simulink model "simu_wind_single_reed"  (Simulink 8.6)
settings: Solver=ode4  StartTime=0.0  StopTime=runtime  FixedStep=1/fs  RelTol=1e-3
PostLoadFcn:
  | , if any(exist('dsrtsu_mdlpostloadfcn', 'file') == [2, 3, 6]), try dsrtsu_mdlpostloadfcn('Execute', bdroot); catch fprintf('Error in PostLoadFcn (dsrtsu_mdlpostloadfcn) for model "%s":
  |  %s
  | ', bdroot, lasterr); end, end,
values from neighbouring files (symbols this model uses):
  an = modal_coeff(:,1)    [hybrid_wind.m]
  gamma_cte = 0.7    [single_reed.m]
  PM = 50    [bowed_string_hyperbolic.m]    (also in lip_reed.m = 20; single_reed.m = 100)
  Qn = modal_coeff(:,3)    [hybrid_wind.m]
  Ts = 25e-6    (= 2.5e-05)    [hybrid_wind.m]    (also in measurements.m)
  wn = modal_coeff(:,2)    [hybrid_wind.m]
  Zc = rho*c/St    (= 2615281.00417)    [hybrid_wind.m]
  zeta = 0.35    [single_reed.m]
undefined symbols (not defined in the file or in its folder): HRreed_G, HRreed_G_zm1, modal_coeff
libraries: simulink x1

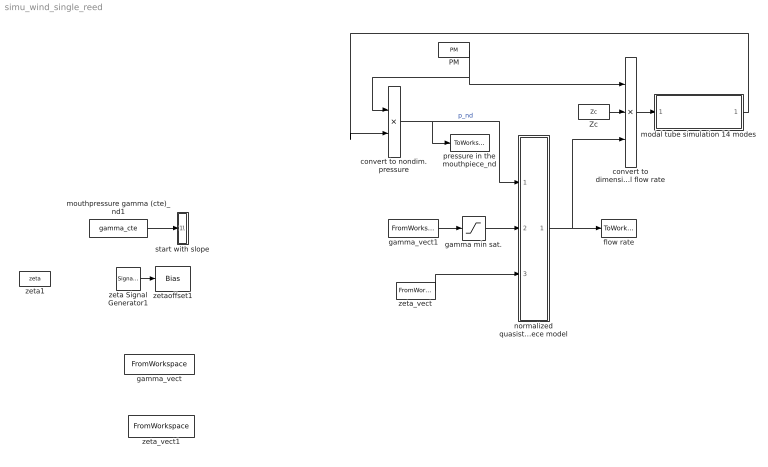
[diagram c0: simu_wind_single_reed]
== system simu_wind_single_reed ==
  PM : Constant  Value=PM
  Zc : Constant  Value=Zc
  convert to dimensional flow rate : Product  Inputs=*/*
  convert to nondim. pressure : Product  Inputs=/*
  flow rate : ToWorkspace  VariableName=q_dl  SaveFormat=Structure  SampleTime=-1
  gamma min sat. : Saturate  UpperLimit=100  LowerLimit=0.3
  gamma_vect : FromWorkspace  VariableName=gamma_envs_all  SampleTime=0
  gamma_vect1 : FromWorkspace  VariableName=gamma_vect  SampleTime=Ts  OutputAfterFinalValue=Setting to zero
  modal tube simulation 14 modes : Subsystem
  mouthpressure gamma (cte)_nd1 : Constant  Value=gamma_cte
  normalized quasistatic mouthpiece model : Subsystem
  pressure in the mouthpiece_nd : ToWorkspace  VariableName=p_dl  SaveFormat=Structure  SampleTime=-1
  start with slope : Subsystem
  zeta Signal Generator1 : SignalGenerator  WaveForm=sawtooth  Amplitude=(0.6-0.1)/2  Frequency=0.2
  zeta1 : Constant  Value=zeta
  zeta_vect : FromWorkspace  VariableName=zeta_vect  SampleTime=Ts  OutputAfterFinalValue=Setting to zero
  zeta_vect1 : FromWorkspace  VariableName=zeta_envs_all_a  SampleTime=0  OutputAfterFinalValue=Setting to zero
  zetaoffset1 : Bias  Bias=0.1+(0.6-0.1)/2
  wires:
  zeta Signal Generator1/1 -> zetaoffset1/1
  Zc/1 -> convert to dimensional flow rate/2
  PM/1 -> convert to nondim. pressure/1, convert to dimensional flow rate/1
  mouthpressure gamma (cte)_nd1/1 -> start with slope/1(gamma_in)
  convert to dimensional flow rate/1 -> modal tube simulation 14 modes/1(flowrate_in)
  modal tube simulation 14 modes/1(p_sim_out) -> convert to nondim. pressure/2
  gamma_vect1/1 -> gamma min sat./1
  gamma min sat./1 -> normalized quasistatic mouthpiece model/2(gamma)
  convert to nondim. pressure/1 -> pressure in the mouthpiece_nd/1, normalized quasistatic mouthpiece model/1(p)  "p_nd"
  normalized quasistatic mouthpiece model/1(q_nd) -> flow rate/1, convert to dimensional flow rate/3
  zeta_vect/1 -> normalized quasistatic mouthpiece model/3(zeta)

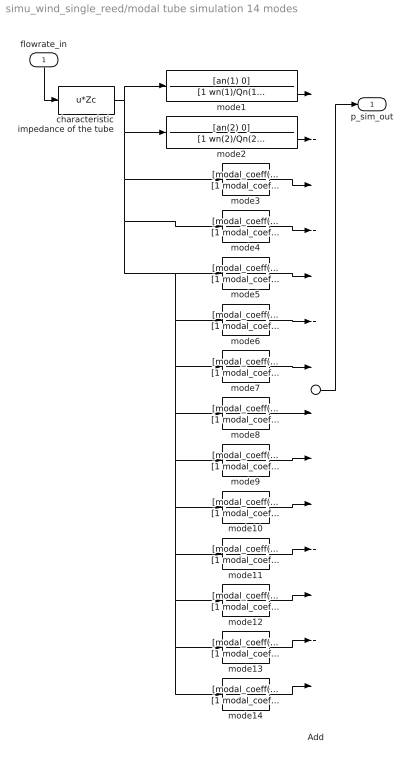
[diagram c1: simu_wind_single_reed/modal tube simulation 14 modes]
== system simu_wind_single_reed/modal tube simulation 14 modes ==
  flowrate_in : Inport
  Add : Sum  Inputs=++++++++++++++
  characteristic impedance of the tube : Fcn  Expr=u*Zc
  mode1 : TransferFcn  Numerator=[an(1) 0]  Denominator=[1 wn(1)/Qn(1) wn(1)^2]
  mode10 : TransferFcn  Numerator=[modal_coeff(10, 1) 0]  Denominator=[1 modal_coeff(10,2)/modal_coeff(10,3) modal_coeff(10,2)^2]
  mode11 : TransferFcn  Numerator=[modal_coeff(11, 1) 0]  Denominator=[1 modal_coeff(11,2)/modal_coeff(11,3) modal_coeff(11,2)^2]
  mode12 : TransferFcn  Numerator=[modal_coeff(12, 1) 0]  Denominator=[1 modal_coeff(12,2)/modal_coeff(12,3) modal_coeff(12,2)^2]
  mode13 : TransferFcn  Numerator=[modal_coeff(13, 1) 0]  Denominator=[1 modal_coeff(13,2)/modal_coeff(13,3) modal_coeff(13,2)^2]
  mode14 : TransferFcn  Numerator=[modal_coeff(14, 1) 0]  Denominator=[1 modal_coeff(14,2)/modal_coeff(14,3) modal_coeff(14,2)^2]
  mode2 : TransferFcn  Numerator=[an(2) 0]  Denominator=[1 wn(2)/Qn(2) wn(2)^2]
  mode3 : TransferFcn  Numerator=[modal_coeff(3, 1) 0]  Denominator=[1 modal_coeff(3,2)/modal_coeff(3,3) modal_coeff(3,2)^2]
  mode4 : TransferFcn  Numerator=[modal_coeff(4, 1) 0]  Denominator=[1 modal_coeff(4,2)/modal_coeff(4,3) modal_coeff(4,2)^2]
  mode5 : TransferFcn  Numerator=[modal_coeff(5, 1) 0]  Denominator=[1 modal_coeff(5,2)/modal_coeff(5,3) modal_coeff(5,2)^2]
  mode6 : TransferFcn  Numerator=[modal_coeff(6, 1) 0]  Denominator=[1 modal_coeff(6,2)/modal_coeff(6,3) modal_coeff(6,2)^2]
  mode7 : TransferFcn  Numerator=[modal_coeff(7, 1) 0]  Denominator=[1 modal_coeff(7,2)/modal_coeff(7,3) modal_coeff(7,2)^2]
  mode8 : TransferFcn  Numerator=[modal_coeff(8, 1) 0]  Denominator=[1 modal_coeff(8,2)/modal_coeff(8,3) modal_coeff(8,2)^2]
  mode9 : TransferFcn  Numerator=[modal_coeff(9, 1) 0]  Denominator=[1 modal_coeff(9,2)/modal_coeff(9,3) modal_coeff(9,2)^2]
  p_sim_out : Outport
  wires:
  flowrate_in/1 -> characteristic impedance of the tube/1
  characteristic impedance of the tube/1 -> mode5/1, mode6/1, mode7/1, mode8/1, mode9/1, mode10/1, mode11/1, mode12/1, mode13/1, mode14/1, mode4/1, mode3/1, mode2/1, mode1/1
  mode1/1 -> Add/1
  Add/1 -> p_sim_out/1
  mode2/1 -> Add/2
  mode3/1 -> Add/3
  mode4/1 -> Add/4
  mode5/1 -> Add/5
  mode6/1 -> Add/6
  mode7/1 -> Add/7
  mode8/1 -> Add/8
  mode9/1 -> Add/9
  mode10/1 -> Add/10
  mode11/1 -> Add/11
  mode12/1 -> Add/12
  mode13/1 -> Add/13
  mode14/1 -> Add/14

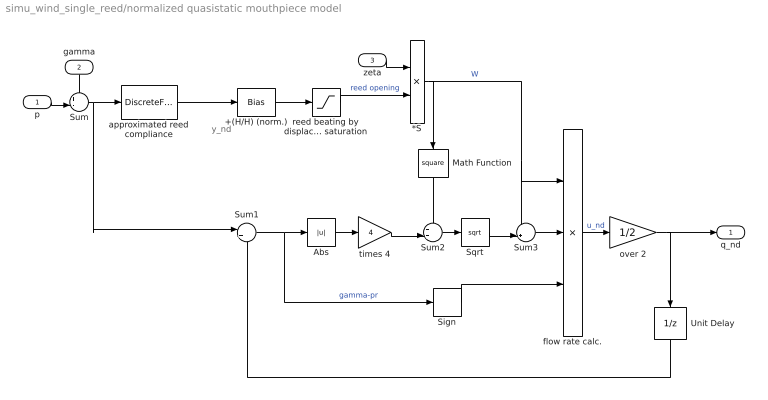
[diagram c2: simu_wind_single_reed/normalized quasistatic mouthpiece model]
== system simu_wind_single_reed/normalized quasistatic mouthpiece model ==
  note: y_nd
  p : Inport
  gamma : Inport  Port=2
  zeta : Inport  Port=3
  *S : Product  Inputs=**
  +(H/H) (norm.) : Bias  Bias=1
  Abs : Abs
  Math Function : Math  Operator=square
  Sign : Signum
  Sqrt : Sqrt
  Sum : Sum  Inputs=+-|
  Sum1 : Sum  Inputs=|++
  Sum2 : Sum  Inputs=++|
  Sum3 : Sum  Inputs=-+|
  Unit Delay : UnitDelay  SampleTime=-1
  approximated reed compliance : DiscreteFilter  Numerator=HRreed_G_zm1.num  Denominator=HRreed_G.den  SampleTime=Ts  a0EqualsOne=on
  flow rate calc. : Product  Inputs=3
  over 2 : Gain  Gain=1/2
  reed beating by displacement saturation : Saturate  UpperLimit=100  LowerLimit=0
  times 4 : Gain  Gain=4
  q_nd : Outport
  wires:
  gamma/1 -> Sum/1
  p/1 -> Sum/2
  zeta/1 -> *S/1
  +(H/H) (norm.)/1 -> reed beating by displacement saturation/1
  Sum2/1 -> Sqrt/1
  Sum1/1 -> Sign/1, Abs/1  "gamma-pr"
  reed beating by displacement saturation/1 -> *S/2  "reed opening"
  Sum/1 -> approximated reed compliance/1, Sum1/1
  *S/1 -> flow rate calc./1, Sum3/1, Math Function/1  "W"
  flow rate calc./1 -> over 2/1  "u_nd"
  Sqrt/1 -> Sum3/2
  Sum3/1 -> flow rate calc./2
  Math Function/1 -> Sum2/1
  Abs/1 -> times 4/1
  times 4/1 -> Sum2/2
  Sign/1 -> flow rate calc./3
  over 2/1 -> q_nd/1, Unit Delay/1
  approximated reed compliance/1 -> +(H/H) (norm.)/1
  Unit Delay/1 -> Sum1/2

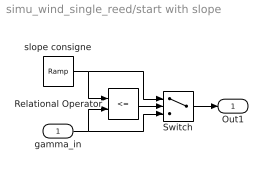
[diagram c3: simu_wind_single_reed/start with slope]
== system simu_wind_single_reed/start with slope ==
  gamma_in : Inport
  Relational Operator : RelationalOperator  Operator=<=  OutDataTypeStr=boolean
  Switch : Switch  Criteria=u2 > Threshold
  slope consigne : simulink/Sources/Ramp  slope=gamma_cte*100  start=0  X0=0
  Out1 : Outport
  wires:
  slope consigne/1 -> Relational Operator/1, Switch/1
  gamma_in/1 -> Relational Operator/2, Switch/3
  Relational Operator/1 -> Switch/2
  Switch/1 -> Out1/1
